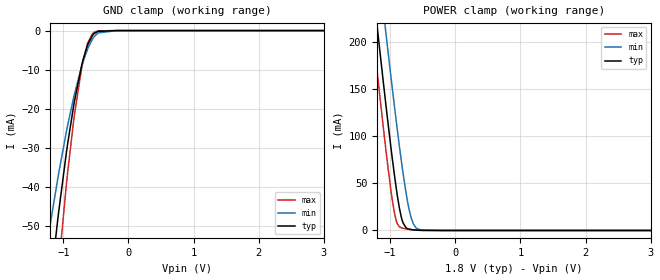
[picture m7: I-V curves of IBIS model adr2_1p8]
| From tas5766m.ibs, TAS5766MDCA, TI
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|   adr2_1p8 Model
[Model]   adr2_1p8
Model_type   Input
Vinl = 0.54
Vinh = 1.26
|   typ   min   max
|   (nom PVT)   (fast PVT)   (slow PVT)
C_comp   6.600e-12   6.468e-12   6.668e-12
[Model spec]
|subparameter
Vinl   0.54   0.486   0.594
Vinh   1.26   1.134   1.386
| Where nom  PVT is Nominal Process, 1.8V, 27C
|   Fast PVT is Strong Process,  1.98V, -40C
|   Slow PVT is Weak Process,   1.62V, 125C
[Voltage Range]   1.8   1.62   1.98
|Junction Temperature
[Temperature Range]   27   125   -40
[Power Clamp Reference]   1.8   1.62   1.98
[GND Clamp Reference]   0   0   0
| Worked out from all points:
|   GND clamp passes 1 mA (typ) near -0.54 V on its own axis
|   POWER clamp passes 1 mA (typ) near -0.68 V on its own axis
[GND Clamp]
|   Voltage   I(typ)   I(min)   I(max)
-1.8V     -252.5mA   -155.8mA   -359.9mA
-1.218V   -68.18mA   -51.5mA    -90.75mA
-1.076V   -47.13mA   -37.04mA   -61.38mA
-952.6mV  -31.24mA   -25.86mA   -39.37mA
-934.2mV  -29.11mA   -24.33mA   -36.44mA
-831.8mV  -18.35mA   -16.47mA   -21.84mA
-716.9mV  -8.869mA   -9.142mA   -9.434mA
-626.4mV  -3.699mA   -4.71mA    -3.198mA
-523.8mV  -726.6uA   -1.504mA   -372.5uA
-465.1mV  -191.4uA   -597.4uA   -66.88uA
-180mV    -64.28nA   -820.8nA   -79.79nA
3.6V      0A         0A         0A
[POWER Clamp]
|   Voltage   I(typ)   I(min)   I(max)
-1.8V     610.8mA    681.1mA    570mA
-1.403V   347mA      421.8mA    301.2mA
-1.192V   211.3mA    287.5mA    163.4mA
-1.101V   154.6mA    231mA      106.6mA
-1.051V   124.5mA    200.6mA    76.9mA
-932.8mV  57.73mA    130.6mA    18.02mA
-856.8mV  23.19mA    88.51mA    3.926mA
-802.8mV  8.103mA    60.94mA    2.322mA
-716.2mV  1.5mA      24.48mA    1.251mA
-644.9mV  681.9uA    7.082mA    634.3uA
-580.3mV  323.9uA    1.677mA    261.2uA
3.6V      0A         0A         0A
